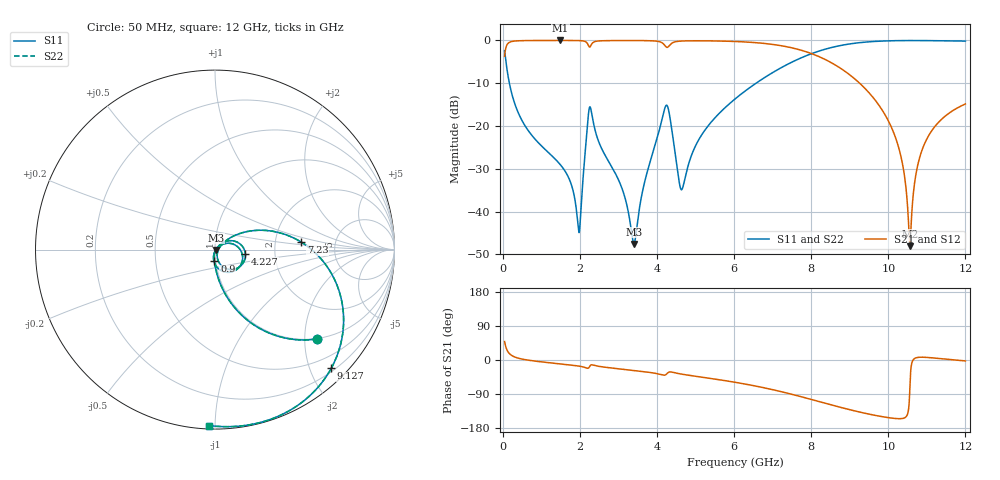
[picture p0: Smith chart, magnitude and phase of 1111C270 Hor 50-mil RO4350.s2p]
# GHz S MA R 50
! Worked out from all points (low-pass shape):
!   11951 points, 50 MHz to 12 GHz, reference 50 ohm
!   highest |S21| = -0.02 dB at 1.498 GHz (marker M1); lowest = -48.1 dB at 10.56 GHz (marker M2)
!   |S21| within 3 dB of the highest: 57.71 MHz to 7.986 GHz (7.928 GHz wide, 197 % of centre)
!   lowest |S11| = -47.6 dB at 3.404 GHz (marker M3), VSWR 1.01, Z = 50.4 - j0.209 ohm
!   |S11| at or under -10 dB: 173.5 MHz to 6.572 GHz (6.398 GHz wide, 190 % of centre)
!   |S22| runs from -47.6 to 0.0 dB; largest |S21 - S12| = 0
!   S11 on the Smith chart (normalised r, x): 50 MHz: 0.98, -2.29; 900 MHz: 0.98, -0.13; 4.227 GHz: 1.41, -0.07; 7.23 GHz: 2.82, +0.31; 9.127 GHz: 0.25, -2.35; 12 GHz: 0.02, -0.97
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0.05  0.756 -41.3  0.6543 48.7  0.6543 48.7  0.756 -41.3
0.231  0.2431 -77.7  0.9696 12.2  0.9696 12.2  0.2431 -77.7
0.9  0.06548 -93.0  0.997 -3.7  0.997 -3.7  0.06548 -93.0
1.498  0.03515 -98.4  0.9981 -10.3  0.9981 -10.3  0.03515 -98.4
1.961  0.006323 -56.1  0.995 -15.9  0.995 -15.9  0.006323 -56.1
2.042  0.01308 29.2  0.9908 -17.3  0.9908 -17.3  0.01308 29.2
2.278  0.1628 -44.9  0.8569 -13.8  0.8569 -13.8  0.1628 -44.9
3.404  0.004173 -29.8  0.9956 -27.5  0.9956 -27.5  0.004173 -29.8
4.034  0.08008 35.8  0.9729 -36.8  0.9729 -36.8  0.08008 35.8
4.227  0.171 -8.0  0.8491 -38.9  0.8491 -38.9  0.171 -8.0
4.643  0.01801 -15.8  0.983 -37.3  0.983 -37.3  0.01801 -15.8
5.122  0.07376 39.2  0.9891 -44.7  0.9891 -44.7  0.07376 39.2
6.025  0.2066 29.2  0.9708 -58.8  0.9708 -58.8  0.2066 29.2
7.23  0.4816 5.1  0.8656 -83.7  0.8656 -83.7  0.4816 5.1
8.017  0.7016 -15.6  0.6983 -104.4  0.6983 -104.4  0.7016 -15.6
9.127  0.9258 -45.6  0.3559 -134.3  0.3559 -134.3  0.9258 -45.6
10.009  0.9879 -64.9  0.113 -152.2  0.113 -152.2  0.9879 -64.9
10.353  0.9944 -71.0  0.03915 -154.6  0.03915 -154.6  0.9944 -71.0
10.56  0.9956 -74.3  0.00394 -73.3  0.00394 -73.3  0.9956 -74.3
10.73  0.9955 -76.9  0.02938 6.1  0.02938 6.1  0.9955 -76.9
10.954  0.9943 -80.0  0.06388 7.1  0.06388 7.1  0.9943 -80.0
12  0.9812 -91.9  0.1808 -2.5  0.1808 -2.5  0.9812 -91.9
